PROGRAM MAIN
VAR
	//输入
	start AT%I* : BOOL;                        //启动按钮
	stop AT%I* : BOOL;                         //停止按钮
	limit_switch_up  AT%I*:BOOL;               //上限位
	limit_switch_down AT%I*:BOOL;              //下限位
	//输出
	solenoid_valve_up AT%Q*:BOOL;              //上行电磁阀
	solenoid_valve_down AT%Q*:BOOL;            //下行电磁阀
	//延时
	delayed_time: TON;                         //下限位延时功能块
	//其他
	state:INT;                                 //状态
	R_TRIG: R_TRIG;                            //检测下限位上升沿信号
	cycle_count:INT;                           //计数
END_VAR

CASE state OF
	0://初始状态
	   solenoid_valve_up := FALSE;                                     //上行电磁阀松开
       solenoid_valve_down := FALSE;	                               //下行电磁阀松开
       cycle_count := 0;                                               // 重置循环次数
	   IF start THEN
	      solenoid_valve_down := TRUE;                                 // 下行电磁阀吸合，气缸下行
          state := 1;                                              
	   END_IF
	1://下行阶段
	    solenoid_valve_down := TRUE;
        IF limit_switch_down THEN                                      //到达下限位
            solenoid_valve_down := FALSE;                              //下行电磁阀松开
        END_IF;
		delayed_time(IN:=limit_switch_down , PT:=T#3S , Q=> , ET=> );  // 启动3秒延时
        IF delayed_time.Q THEN
            solenoid_valve_up := TRUE;                                 // 上行电磁阀吸合
            state := 2;                                                                                                                   
        END_IF;
    2://上行阶段
	  solenoid_valve_up := TRUE;
	  R_TRIG(CLK:=limit_switch_UP , Q=> );
      IF R_TRIG.Q THEN
         cycle_count := cycle_count + 1;                              // 循环次数+1
         solenoid_valve_up := FALSE;                                  // 上行电磁阀松开
         state := 1;                                                  // 切换回下行状态（开始下一次循环）
      END_IF;
      IF cycle_count >= 3 THEN                                        //清洗次数达到3次回到初始位
         state := 0;
      END_IF; 
    3://按下停止按钮后强制上行到上限位
      IF limit_switch_UP THEN                                       
         solenoid_valve_up := FALSE;                                 // 松开上行电磁阀
         state := 0;                                                 // 回到初始状态（停止所有动作）
      END_IF;  
END_CASE

IF stop THEN                                                         //按下停止按钮
   solenoid_valve_up := TRUE;                                        //上行电磁阀吸合
   solenoid_valve_down := FALSE;                                     //下行电磁阀松开
   state:=3;
END_IF

END_PROGRAM
